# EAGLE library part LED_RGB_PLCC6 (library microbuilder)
RGB LED Cree CLV6A-FKB - Digikey: CLV6A-FKB-CK1P1G1BB7R3R3TR-ND DC Foreward Current: 20mA Foreward Voltage: R = 2.0, G = 3.2, B = 3.2 Viewing Angle: 120°
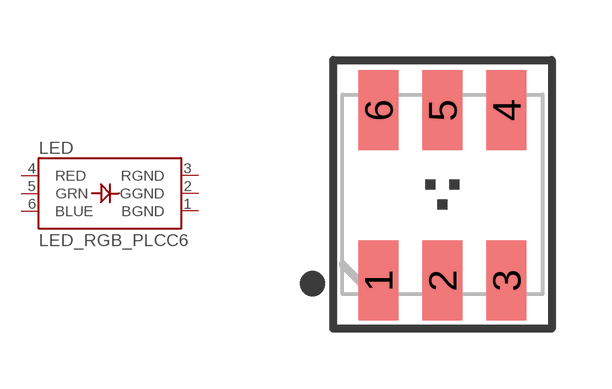
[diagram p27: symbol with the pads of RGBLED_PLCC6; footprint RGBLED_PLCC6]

Designator prefix LED

## LED_RGB_PLCC6CREE-CLV6A  [RGBLED_PLCC6]
1  BGND  pwr
2  GGND  pwr
3  RGND  pwr
4  RED
5  GRN
6  BLUE

## Footprint RGBLED_PLCC6 (pad centres in mm)
RGB LED PLCC-6 5.0mm x 5.0mm 1.5mm Pitch
smd 1 x 2: 1 -1.6,-2.158; 2 0,-2.158; 3 1.6,-2.158; 4 1.6,2.108; 5 0,2.108; 6 -1.6,2.108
